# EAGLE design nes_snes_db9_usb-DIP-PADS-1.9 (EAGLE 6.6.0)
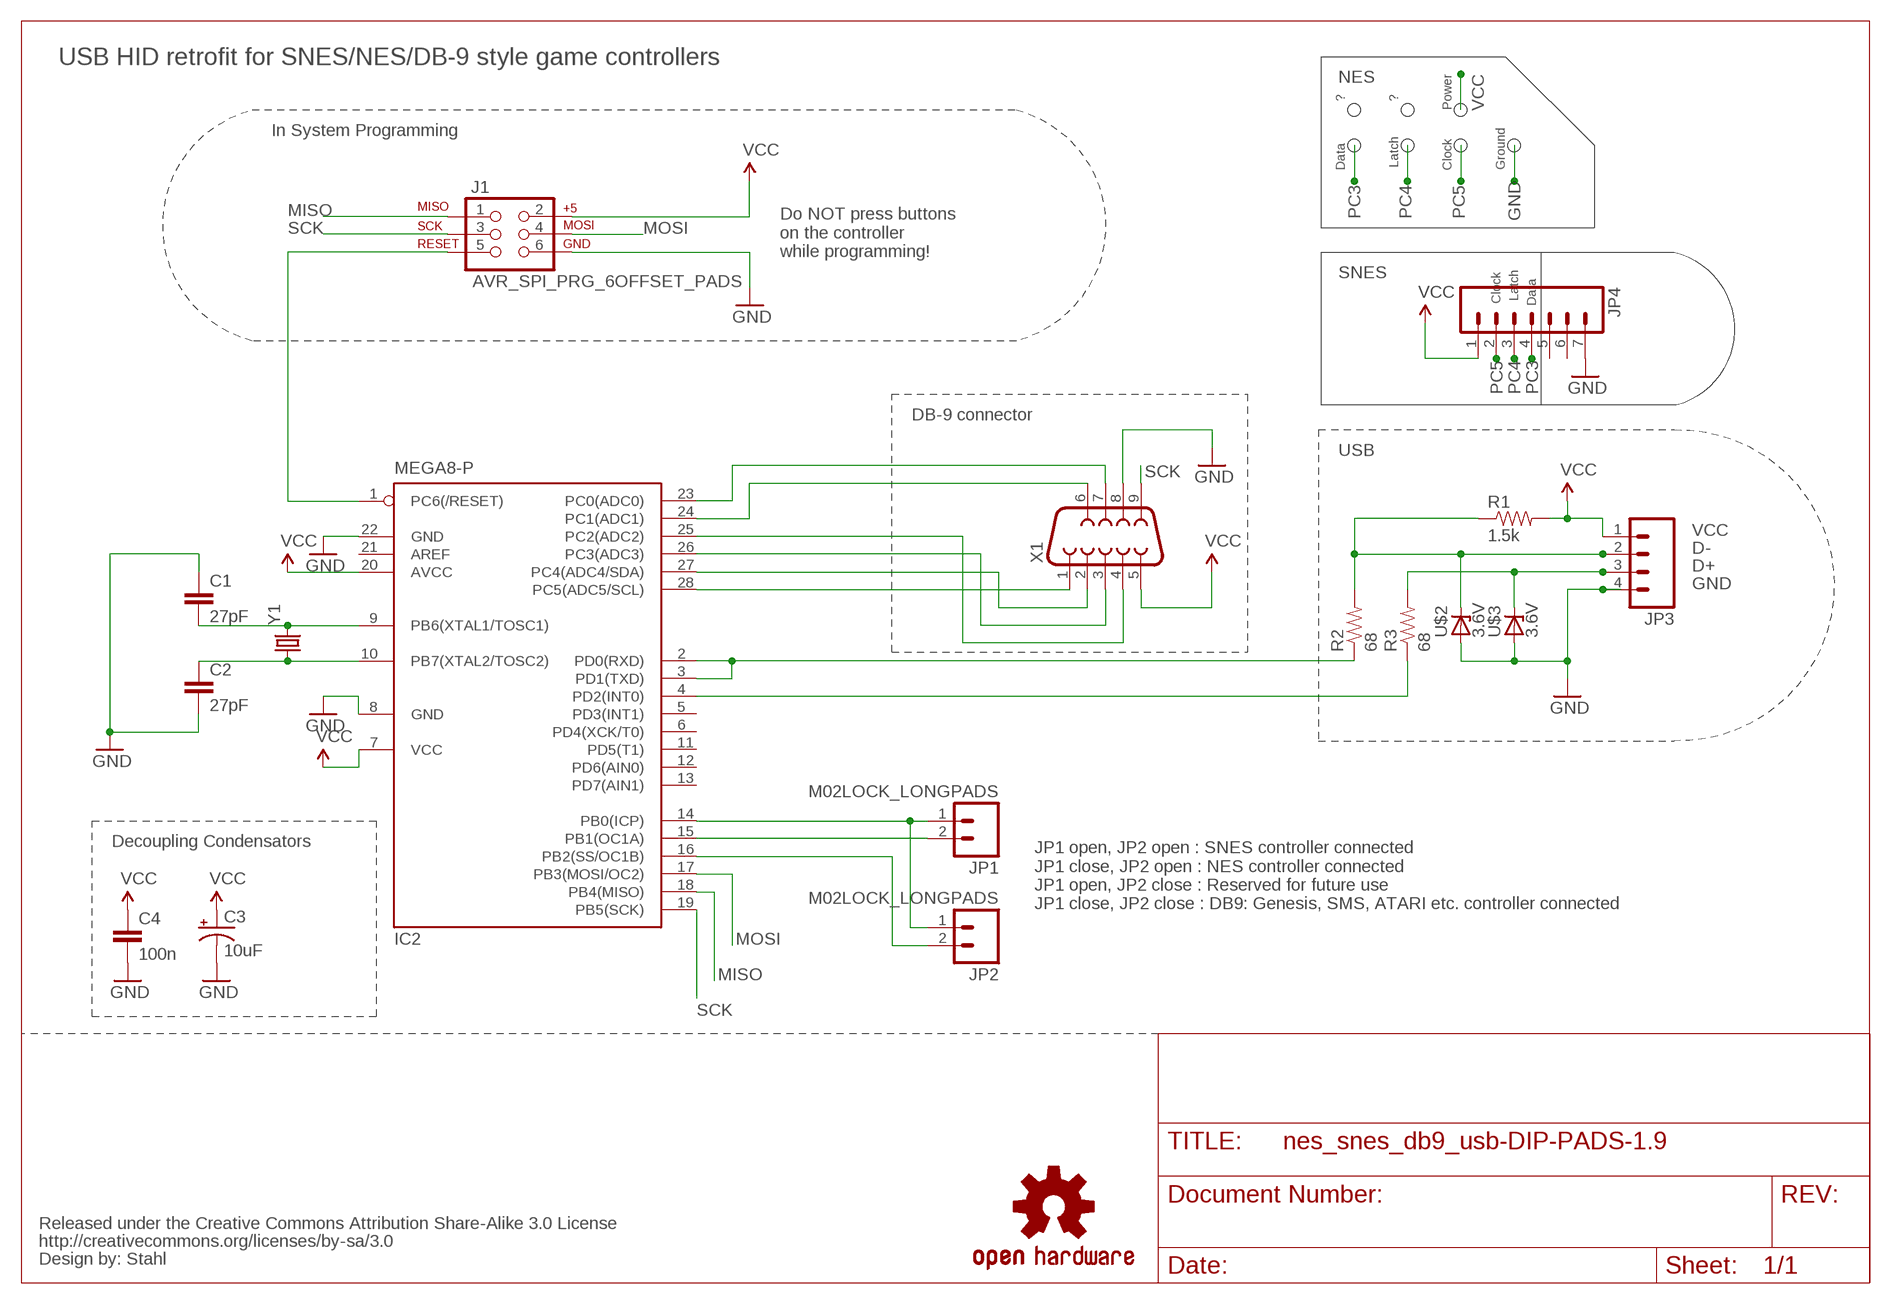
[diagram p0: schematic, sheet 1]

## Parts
C1  27pF  CAP1206  [1206]
C2  27pF  CAP1206  [1206]
C3  10uF  CPOL-USB  [PANASONIC_B]
C4  100n  CAP1206  [1206]
CC_TEXT1  CREATIVE_COMMONS  [CREATIVE_COMMONS]
IC2  MEGA8-P  [DIL28-3]
J1  AVR_SPI_PRG_6OFFSET_PADS  [2X3_OFFSET]
JP1  M02LOCK_LONGPADS  [1X02_LOCK_LONGPADS]
JP2  M02LOCK_LONGPADS  [1X02_LOCK_LONGPADS]
JP3  M04LONGPADS  [1X04_LONGPADS]
JP4  M07  [1X07]
LOGO1  OSHW-LOGOL  [OSHW-LOGO-L]
R1  1.5k  RESISTOR1206  [1206]
R2  68  RESISTOR1206  [1206]
R3  68  RESISTOR1206  [1206]
U$2  3.6V  ZENER-DIODESOD80C  [SOD80C]
U$3  3.6V  ZENER-DIODESOD80C  [SOD80C]
X1  DB9MALE  [DB9_MALE]
Y1  CRYSTALSMD  [HC49UP]

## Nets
D+: JP3.3 R3.2 U$3.C
D-: JP3.2 R1.1 R2.2 U$2.C
GND: C1.1 C2.2 C3.- C4.2 IC2.8(GND) IC2.22(GND) J1.6 JP3.4 JP4.7 U$2.A U$3.A X1.8
MISO: IC2.18(PB4(MISO)) J1.1
MOSI: IC2.17(PB3(MOSI/OC2)) J1.4
N$2: C1.2 IC2.9(PB6(XTAL1/TOSC1)) Y1.2
N$3: C2.1 IC2.10(PB7(XTAL2/TOSC2)) Y1.1
N$6: IC2.14(PB0(ICP)) JP1.1 JP2.1
N$7: IC2.15(PB1(OC1A)) JP1.2
N$8: IC2.16(PB2(SS/OC1B)) JP2.2
N$10: IC2.2(PD0(RXD)) IC2.3(PD1(TXD)) R2.1
N$12: IC2.4(PD2(INT0)) R3.1
PC0: IC2.23(PC0(ADC0)) X1.7
PC1: IC2.24(PC1(ADC1)) X1.6
PC2: IC2.25(PC2(ADC2)) X1.4
PC3: IC2.26(PC3(ADC3)) JP4.4 X1.3
PC4: IC2.27(PC4(ADC4/SDA)) JP4.3 X1.2
PC5: IC2.28(PC5(ADC5/SCL)) JP4.2 X1.1
RESET: IC2.1(PC6(/RESET)) J1.5
SCK: IC2.19(PB5(SCK)) J1.3 X1.9
VCC: C3.+ C4.1 IC2.7(VCC) IC2.20(AVCC) J1.2 JP3.1 JP4.1 R1.2 X1.5
Unconnected: IC2.5(PD3(INT1)) IC2.6(PD4(XCK/T0)) IC2.11(PD5(T1)) IC2.12(PD6(AIN0)) IC2.13(PD7(AIN1)) IC2.21(AREF) JP4.5 JP4.6

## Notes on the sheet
- USB HID retrofit for SNES/NES/DB-9 style game controllers
- NES
- ? | ?
- Power
- Ground
- In System Programming | Latch | Clock
- Data
- Do NOT press buttons
  on the controller
  while programming!
- Clock | Latch
- SNES | Data
- DB-9 connector
- USB
- Decoupling Condensators
- JP1 open, JP2 open : SNES controller connected
  JP1 close, JP2 open : NES controller connected
  JP1 open, JP2 close : Reserved for future use
  JP1 close, JP2 close : DB9: Genesis, SMS, ATARI etc. controller connected

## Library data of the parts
C1 C2 C4 = SparkFun-Capacitors:CAP: Capacitor
C3 = adafruit:CPOL-US: POLARIZED CAPACITOR, American symbol
CC_TEXT1 = SparkFun-Aesthetics:CREATIVE_COMMONS: Creative Commons License summary
IC2 = atmel:MEGA8-P: MICROCONTROLLER 8 Kbytes FLASH, 1 kbytes SRAM, 512 bytes EEPROM, USART, 4-channel 10 bit ADC, 2-channel 8 bit ADC Pin compatible with Atmega48, ATMega88, ATMega168 Source: avr.lbr; OC_FARNELL: unknown; OC_NEWARK: unknown
J1 = SparkFun-Connectors:AVR_SPI_PRG_6: AVR ISP 6 Pin This is the reduced ISP connector for AVR programming. Common on Arduino. This footprint will take up less PCB space and can be used with a 10-pin to 6-pin adapter such as SKU: BOB-08508
JP1 JP2 = SparkFun-Connectors:M02: Standard 2-pin 0.1" header. Use with
JP3 = SparkFun-Connectors:M04: Header 4 Standard 4-pin 0.1" header. Use with straight break away headers (SKU : PRT-00116), right angle break away headers (PRT-00553), swiss pins (PRT-00743), machine pins (PRT-00117), and female headers (PRT-00115). Molex polarized connector foot print use with SKU : PRT-08231 with associated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
JP4 = SparkFun-Connectors:M07: Header 7 Standard 7-pin 0.1" header. Use with straight break away headers (SKU : PRT-00116), right angle break away headers (PRT-00553), swiss pins (PRT-00743), machine pins (PRT-00117), and female headers (PRT-00115). NOTES ON THE VARIANTS LOCK and LOCK_LONGPADS... This footprint was designed to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
LOGO1 = SparkFun-Aesthetics:OSHW-LOGO: Open Source Hardware Logo This logo indicates the piece of hardware it is found on incorporates a OSHW license and/or adheres to the definition of open source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
R1-R3 = SparkFun-Resistors:RESISTOR: Resistor
U$2 U$3 = diode:ZENER-DIODE: Z-Diode
X1 = SparkFun-Connectors:DB9: DB9 Connector Standard DB9 (D-Sub 9) serial connector. Can be used for CAN bus as well as RS485 and RS232. Footprint production proven. Spark Fun Electronics SKU : PRT-00429
Y1 = SparkFun-FreqCtrl:CRYSTAL: Various standard crystals. Proven footprints. Spark Fun Electronics SKU : COM-00534

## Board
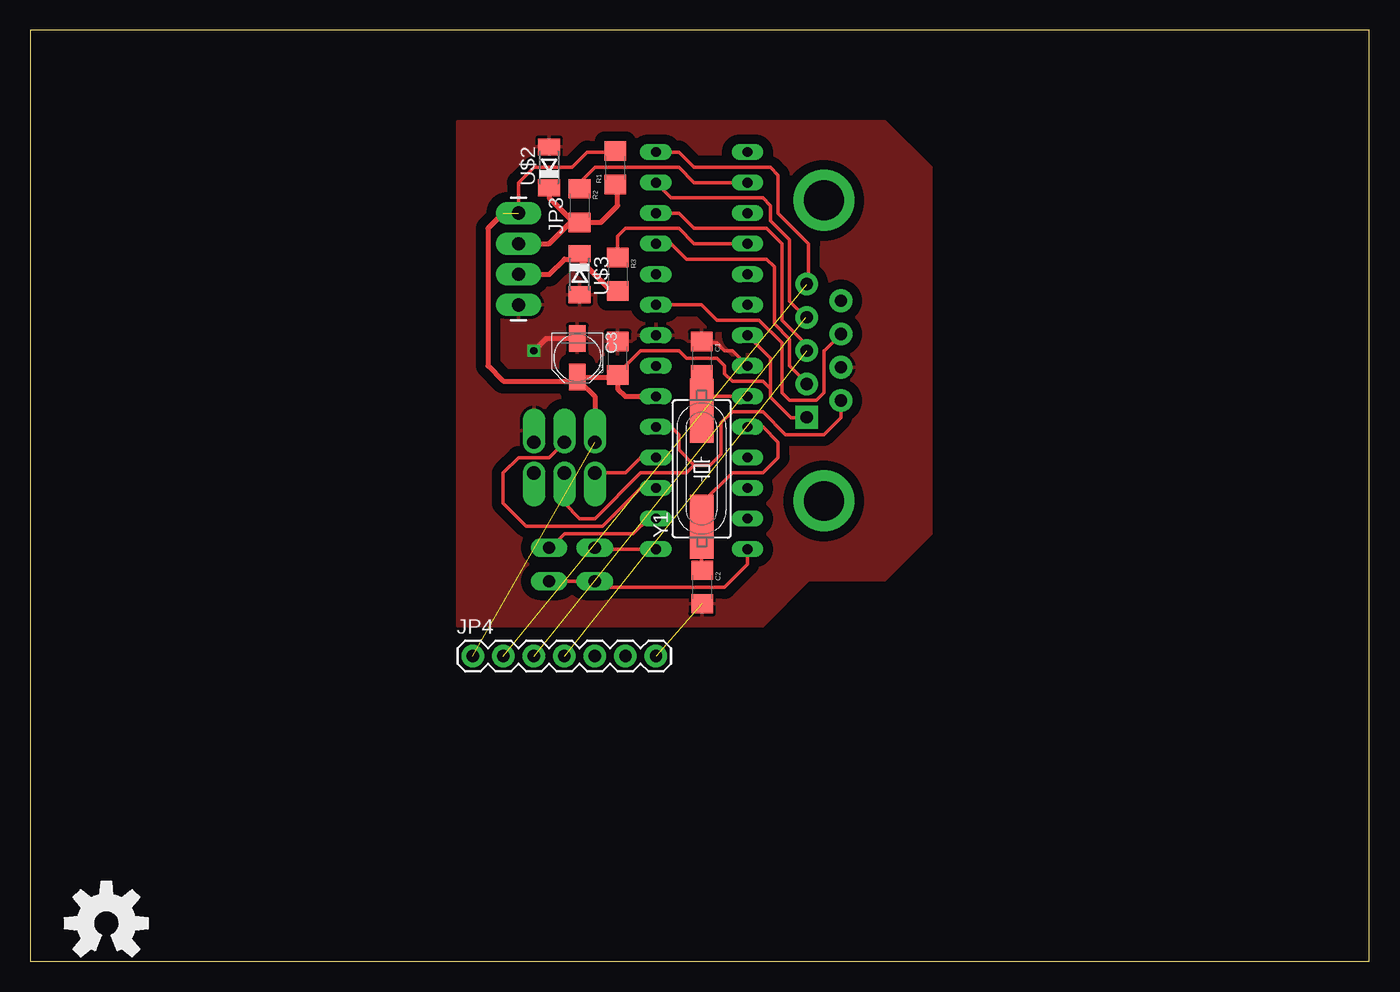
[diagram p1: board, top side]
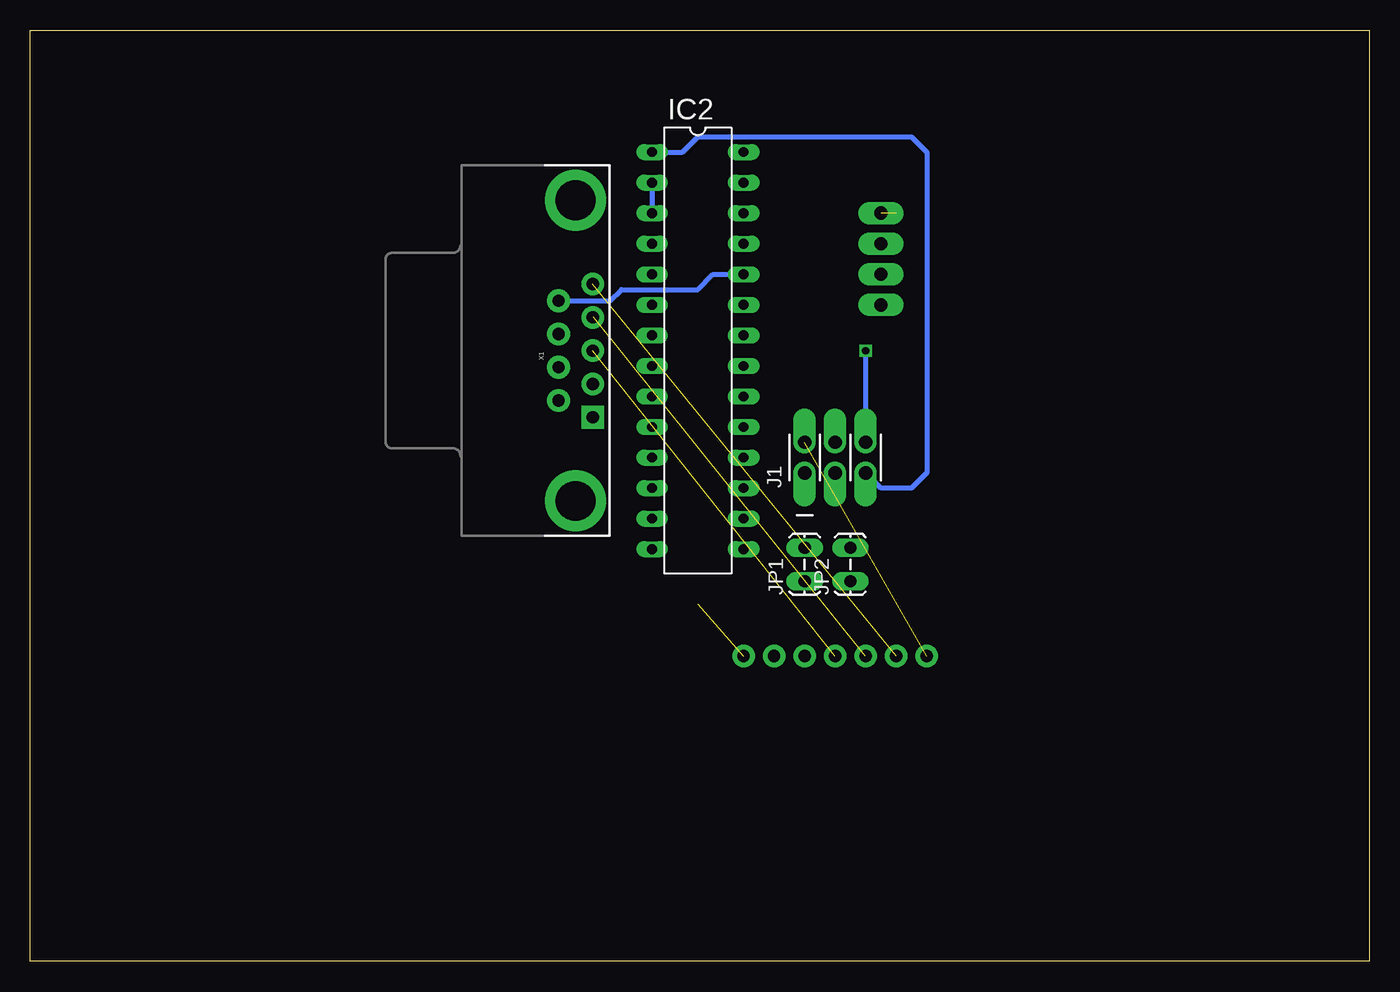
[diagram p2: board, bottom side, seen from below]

Size 111.43 x 77.46 mm. Coordinates in mm from the lower left corner, seen from the top.
Outline: 0,0 111.43,0 111.43,77.46 0,77.46 0,0
Copper layers (1*16): Top 0.035mm / dielectric 1.5mm / Bottom 0.035mm
Design rules "default": minimum track width 10mil, minimum drill 24mil, track to track 8mil, track to pad 8mil, pad to pad 8mil, via to via 8mil, smd to smd 8mil, copper to edge 40mil, drill to drill 8mil, minimum pad ring 10mil, minimum via ring 8mil, stop-mask expansion 4mil, vias tented up to drill 0mil, thermal gap 10mil

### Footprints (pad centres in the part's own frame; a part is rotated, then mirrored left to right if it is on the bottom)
1206 = smd 1.6 x 1.8: 1 -1.4,0; 2 1.4,0
PANASONIC_B = smd 2.2 x 1.4: + 1.6,0; - -1.6,0
DIL28-3 = drill 0.813 long: 1 -16.51,-3.81; 2 -13.97,-3.81; 3 -11.43,-3.81; 4 -8.89,-3.81; 5 -6.35,-3.81; 6 -3.81,-3.81; 7 -1.27,-3.81; 8 1.27,-3.81; 9 3.81,-3.81; 10 6.35,-3.81; 11 8.89,-3.81; 12 11.43,-3.81; 13 13.97,-3.81; 14 16.51,-3.81; 15 16.51,3.81; 16 13.97,3.81; 17 11.43,3.81; 18 8.89,3.81; 19 6.35,3.81; 20 3.81,3.81; 21 1.27,3.81; 22 -1.27,3.81; 23 -3.81,3.81; 24 -6.35,3.81; 25 -8.89,3.81; 26 -11.43,3.81; 27 -13.97,3.81; 28 -16.51,3.81
2X3_OFFSET = drill 1.118 pad 1.88 offset: 1 -2.54,-1.27; 2 -2.54,1.27; 3 0,-1.27; 4 0,1.27; 5 2.54,-1.27; 6 2.54,1.27
1X02_LOCK_LONGPADS = drill 1.016 long: 1 -0.127,0; 2 2.667,0
1X04_LONGPADS = drill 1.118 pad 1.88 long: 1 0,0; 2 2.54,0; 3 5.08,0; 4 7.62,0
1X07 = drill 1.016 pad 1.88: 1 0,0; 2 2.54,0; 3 5.08,0; 4 7.62,0; 5 10.16,0; 6 12.7,0; 7 15.24,0
SOD80C = smd 1.4 x 1.8: A 1.7,0; C -1.7,0
DB9_MALE = drill 1.016 pad 1.88: 1 5.54,-1.42; 2 2.77,-1.42; 3 0,-1.42; 4 -2.77,-1.42; 6 4.15,1.42; 7 1.38,1.42; 8 -1.38,1.42; 9 -4.15,1.42 | drill 1.016 pad 1.88 square: 5 -5.54,-1.42 | drill 3.302 pad 5.08: G1 -12.5,0; G2 12.5,0
HC49UP = smd 5.334 x 1.93: 1 -4.826,0; 2 4.826,0

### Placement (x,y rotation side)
C1  55.88,50.16 270 top
C2  55.91,31.14 270 top
C3  45.52,50.2 270 top
C4  48.9,50.16 90 top
CC_TEXT1  22.86,2.54 0 top
IC2  55.88,50.8 270 bottom
J1  44.45,41.91 0 bottom
JP1  46.99,31.75 90 bottom
JP2  43.18,31.75 90 bottom
JP3  40.64,62.23 270 top
JP4  36.83,25.4 0 top
LOGO1  6.35,3.17 0 top
R1  48.7,66.01 90 top
R2  45.72,62.87 270 top
R3  48.9,57.15 270 top
U$2  43.18,66.04 90 top
U$3  45.72,57.15 270 top
X1  66.04,50.8 90 bottom
Y1  55.88,40.97 90 top

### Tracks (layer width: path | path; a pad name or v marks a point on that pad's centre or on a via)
D+
  Top 0.406: JP3.3 43.18,57.15 44.45,58.42 45.29,58.42 U$3.C 45.72,58.42 48.26,55.88 48.77,55.88 R3.2
D-
  Top 0.305: R2.2 46.54,61.46
  Top 0.406: R1.1 48.9,64.41 48.9,62.87 47.49,61.46 R2.2 45.59,61.59 45.09,61.59 | U$2.C 43.18,63.5 45.09,61.59 | JP3.2 43.18,59.69 45.09,61.59
GND  (via drill 0.6 pad 0.3)  (1 unrouted)
  Top 0.305: IC2.8 58.42,50.8 57.78,50.8 57.15,51.44 56.01,51.44 C1.1
  Top 0.406: C3.- 42.91,51.8 v41.91,50.8
  Bottom 0.406: v41.91,50.8 J1.6
  pour Top (isolate 0.813): 35.56,69.85 71.12,69.85 74.93,66.04 74.93,35.56 71.12,31.75 64.77,31.75 60.96,27.94 35.56,27.94
MISO
  Top 0.305: J1.1 49.53,40.64 50.8,41.91 IC2.18
MOSI
  Top 0.305: J1.4 43.18,41.91 40.64,41.91 39.37,40.64 39.37,38.1 41.27,36.2 47.62,36.2 50.8,39.37 IC2.17
N$2
  Top 0.305: 55.88,46.99 C1.2 | Y1.2 55.88,46.99 | 55.88,46.99 IC2.9
N$3
  Top 0.305: IC2.10 60.96,44.45 62.23,43.18 62.23,41.91 60.96,40.64 58.42,40.64 55.88,38.1 Y1.1 55.88,32.58 C2.1
N$6
  Top 0.305: JP2.1 JP1.1 47.5,31.11 57.78,31.11 59.69,33.02 IC2.14
N$7
  Top 0.305: JP1.2 46.86,34.42 46.99,34.29 IC2.15
N$8
  Top 0.305: JP2.2 43.31,34.42 44.45,35.56 50.16,35.56 51.44,36.83 IC2.16
N$10
  Top 0.305: IC2.2 55.24,64.77 53.98,66.04 46.99,66.04 45.72,64.77 R2.1
  Bottom 0.406: IC2.2 IC2.3
N$12
  Top 0.305: R3.1 49.53,58.42 48.9,58.42 48.9,60.32 49.53,60.96 53.98,60.96 55.24,59.69 IC2.4
PC0
  Top 0.305: IC2.23 55.88,54.61 57.15,53.34 60.64,53.34 62.55,51.44 62.55,47.31 63.18,46.67 65.41,46.67 66.04,47.31 66.04,50.8 66.08,50.8 X1.7
PC1
  Bottom 0.406: X1.6 63.16,54.95 62.23,55.88 55.88,55.88 54.61,57.15 IC2.24
PC2
  Top 0.305: X1.4 64.36,48.35 63.18,49.53 63.18,51.75 61.91,53.02 61.91,57.78 61.28,58.42 54.61,58.42 53.34,59.69 IC2.25
PC3  (1 unrouted)
  Top 0.305: X1.3 64.67,51.22 62.55,53.34 62.55,59.69 61.28,60.96 55.24,60.96 53.98,62.23 IC2.26
PC4  (1 unrouted)
  Top 0.305: X1.2 64.54,53.57 63.18,54.93 63.18,60.01 61.59,61.59 61.59,62.87 60.96,63.5 53.34,63.5 IC2.27
PC5  (1 unrouted)
  Top 0.305: X1.1 64.94,56.34 64.77,56.52 64.77,59.69 62.23,62.23 62.23,65.41 61.59,66.04 55.24,66.04 53.98,67.31 IC2.28
RESET
  Bottom 0.406: IC2.1 57.15,67.31 55.88,68.58 38.1,68.58 36.83,67.31 36.83,40.64 38.1,39.37 40.64,39.37 J1.5
SCK
  Top 0.305: X1.9 67.46,45.23 66.04,43.81 62.87,43.81 60.96,45.72 58.42,45.72 57.5,44.8 57.5,42.2 56.58,41.27 55.24,41.27 | J1.3 44.45,38.1 45.72,36.83 46.99,36.83 50.8,40.64 54.61,40.64 55.24,41.27 | IC2.19 53.34,44.45 53.98,43.81 53.98,42.55 55.24,41.27
VCC  (2 unrouted)
  Top 0.305: 61.59,47.62 61.59,50.16 IC2.7 | 61.59,47.62 60.96,48.26 58.42,48.26 57.78,48.89 57.78,49.53 57.15,50.16 54.61,50.16 53.98,50.8 50.8,50.8 48.9,48.89 | 61.59,47.62 61.59,46.91 63.3,45.2 64.56,45.2 X1.5 64.56,45.26 | R1.2 48.36,67.41 | 48.6,67.31 46.35,67.31 45.09,66.04 41.91,66.04 40.64,64.77 JP3.1
  Top 0.406: 48.6,67.31 R1.2 | 39.37,62.23 38.1,60.96 38.1,49.53 39.37,48.26 45.18,48.26 | 45.18,48.26 C3.+ 48.73,48.6 C4.1 | C4.1 48.9,48.89 | C4.1 48.9,47.62 49.53,46.99 IC2.20 | 45.18,48.26 45.72,48.26 46.99,46.99 J1.2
